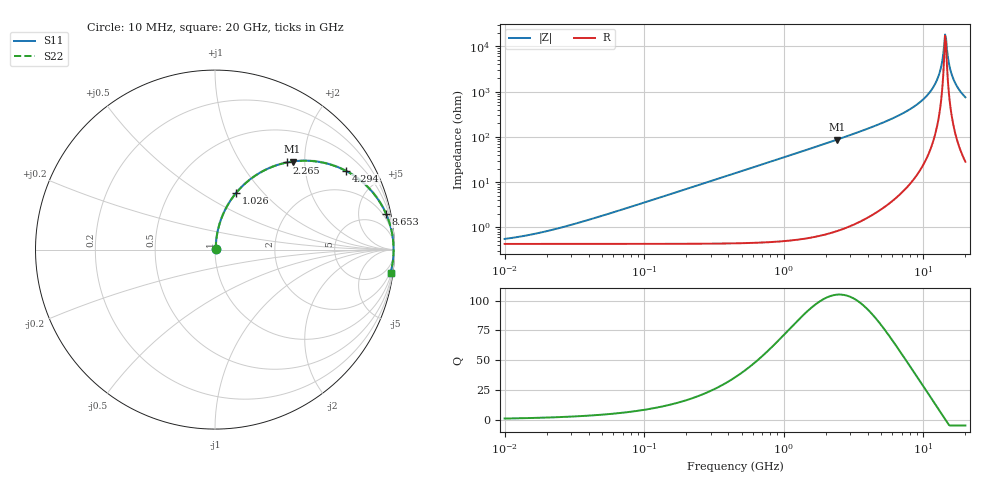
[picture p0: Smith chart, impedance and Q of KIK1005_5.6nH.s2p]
!version-3
!date-01.2023
!Series
# Hz S RI R 50
!Freq ReS11 ImS11 ReS21 ImS21 ReS12 ImS12 ReS22 ImS22
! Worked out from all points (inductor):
!   500 points, 10 MHz to 20 GHz, reference 50 ohm
!   read as one part in series: L = 5.6 nH near 37.06 MHz
!   highest Q = 105 at 2.407 GHz (marker M1), where L = 5.76 nH
!   self-resonance near 14.31 GHz
!   S11 on the Smith chart (normalised r, x): 10 MHz: 1.01, +0.01; 1.026 GHz: 1.01, +0.73; 2.265 GHz: 1.02, +1.63; 4.294 GHz: 1.04, +3.32; 8.653 GHz: 1.24, +9.54; 20 GHz: 2, -15
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1e7  0.00431 0.00349  0.9957 -0.00349  0.9957 -0.00349  0.00431 0.00349
1.783943e7  0.00434 0.00622  0.9957 -0.00622  0.9957 -0.00622  0.00434 0.00622
3.59488e7  0.00446 0.0125  0.9955 -0.0125  0.9955 -0.0125  0.00446 0.0125
1.272781e8  0.00629 0.0443  0.9937 -0.0443  0.9937 -0.0443  0.00629 0.0443
4.506326e8  0.0287 0.1535  0.9713 -0.1535  0.9713 -0.1535  0.0287 0.1535
1.025766e9  0.1197 0.3178  0.8803 -0.3178  0.8803 -0.3178  0.1197 0.3178
1.595481e9  0.2465 0.4257  0.7535 -0.4257  0.7535 -0.4257  0.2465 0.4257
2.264871e9  0.4013 0.4854  0.5987 -0.4854  0.5987 -0.4854  0.4013 0.4854
2.407158e9  0.4322 0.4906  0.5678 -0.4906  0.5678 -0.4906  0.4322 0.4906
4.294233e9  0.7312 0.4377  0.2688 -0.4377  0.2688 -0.4377  0.7312 0.4377
5.648861e9  0.8432 0.3566  0.1568 -0.3566  0.1568 -0.3566  0.8432 0.3566
8.653445e9  0.9533 0.1986  0.0467 -0.1986  0.0467 -0.1986  0.9533 0.1986
1.071034e10  0.9813 0.1153  0.0187 -0.1153  0.0187 -0.1153  0.9813 0.1153
1.228403e10  0.9911 0.0616  0.00894 -0.0616  0.00894 -0.0616  0.9911 0.0616
1.325614e10  0.9939 0.0317  0.0061 -0.0317  0.0061 -0.0317  0.9939 0.0317
1.408894e10  0.9949 0.0079  0.00512 -0.0079  0.00512 -0.0079  0.9949 0.0079
1.430519e10  0.9949 0.00194  0.00506 -0.00194  0.00506 -0.00194  0.9949 0.00194
1.47477e10  0.9949 -0.00999  0.00515 0.00999  0.00515 0.00999  0.9949 -0.00999
1.543725e10  0.9942 -0.0279  0.00581 0.0279  0.00581 0.0279  0.9942 -0.0279
1.640708e10  0.9923 -0.0517  0.00771 0.0517  0.00771 0.0517  0.9923 -0.0517
1.797724e10  0.9872 -0.0875  0.0128 0.0875  0.0128 0.0875  0.9872 -0.0875
2e10  0.9779 -0.1293  0.0221 0.1293  0.0221 0.1293  0.9779 -0.1293
